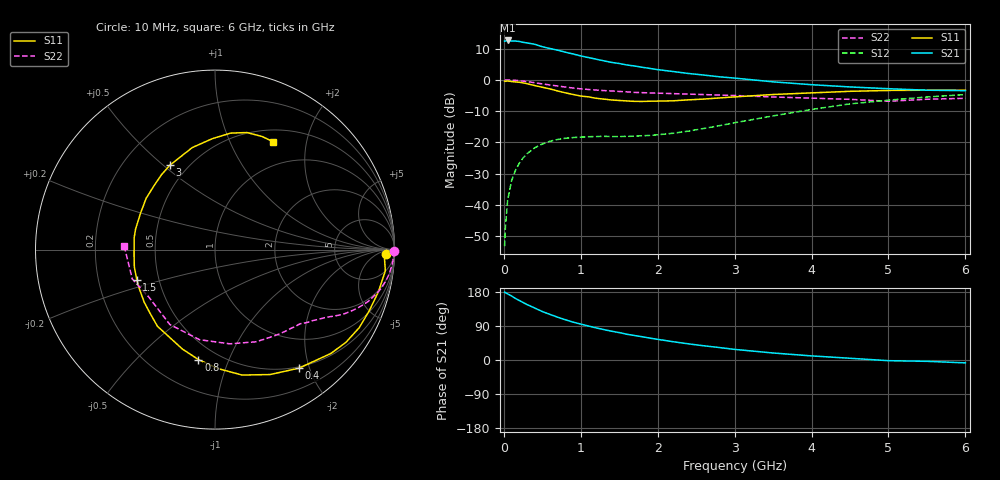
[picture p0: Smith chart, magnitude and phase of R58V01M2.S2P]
! SIEMENS Small Signal Semiconductors
! BFR183
! Si NPN RF Bipolar Junction Transistor in SOT23
! VCE = 8 V  IC = 1.2 mA
! Common Emitter S-Parameters:  May  1996
# GHz  S  MA  R  50
!  f  S11  S21  S12  S22
! GHz  MAG  ANG  MAG  ANG  MAG  ANG  MAG  ANG
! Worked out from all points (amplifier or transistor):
!   36 points, 10 MHz to 6 GHz, reference 50 ohm
!   highest |S21| = 12.6 dB at 50 MHz (marker M1)
!   |S21| within 3 dB of that: start of sweep to 680.6 MHz
!   unconditionally stable (mu >= 1): 1.625 GHz to 2.917 GHz
!   at 250 MHz: K = 0.17, MSG = 18.5 dB, |S12| = -24.9 dB
!   at 1.4 GHz: K = 0.88, MSG = 11.9 dB, |S12| = -18.1 dB
!   at 6 GHz: K = 0.93, MSG = 0.6 dB, |S12| = -4.7 dB
!   S11 on the Smith chart (normalised r, x): 10 MHz: 33, -17; 400 MHz: 0.48, -1.84; 800 MHz: 0.39, -0.78; 1.5 GHz: 0.37, -0.16; 3 GHz: 0.40, +0.53; 6 GHz: 0.65, +1.47
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0.01  0.9529 -1.4  4.137 179.2  0.0022 85.5  0.9973 -0.5
0.02  0.946 -3.2  4.159 177.6  0.0044 88.5  0.9937 -1.0
0.05  0.9564 -7.1  4.252 174.4  0.0121 85.8  0.9958 -2.7
0.1  0.9403 -14.4  4.162 169.0  0.0242 81.3  0.9885 -5.3
0.15  0.9247 -21.6  4.162 162.5  0.0355 77.3  0.9802 -8.0
0.2  0.9138 -28.4  4.101 157.1  0.0464 73.6  0.9672 -10.4
0.3  0.8668 -41.9  3.889 146.4  0.0658 66.1  0.9365 -14.9
0.4  0.8094 -54.7  3.697 137.3  0.0818 59.2  0.899 -18.9
0.5  0.7608 -66.2  3.381 127.9  0.0944 53.3  0.8599 -22.2
0.7  0.663 -88.6  2.975 112.9  0.1114 44.7  0.7964 -27.0
0.8  0.6195 -98.6  2.763 106.2  0.1164 41.3  0.766 -28.8
0.9  0.5832 -108.1  2.586 100.0  0.1196 39.1  0.738 -30.5
1.1  0.5341 -126.9  2.268 89.7  0.1233 36.0  0.7007 -33.5
1.3  0.4915 -143.3  2.01 80.3  0.1252 34.6  0.6729 -36.0
1.5  0.4673 -158.7  1.821 72.3  0.1241 35.5  0.6511 -38.7
1.9  0.4552 171.8  1.52 57.7  0.1293 41.8  0.6179 -44.2
2.2  0.4618 154.0  1.356 48.3  0.14 47.5  0.6019 -48.8
3  0.5333 118.1  1.065 28.0  0.2059 56.6  0.5619 -66.1
3.5  0.5822 102.6  0.928 18.5  0.2652 55.1  0.5314 -81.1
4.5  0.6547 82.4  0.769 4.6  0.4124 43.5  0.4874 -121.1
5.5  0.6825 67.4  0.682 -3.5  0.5318 27.3  0.4893 -160.5
6  0.6829 61.6  0.671 -7.6  0.5806 17.4  0.5065 177.5
